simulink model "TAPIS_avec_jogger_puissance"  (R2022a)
settings: Solver=ode23t  StartTime=0.0  StopTime=30  RelTol=1e-3  EnableMultiTasking=on
libraries: fl_lib x15, nesl_utility x8, fl_ps_legacy_lib x1, simulink x1, ee_lib x1

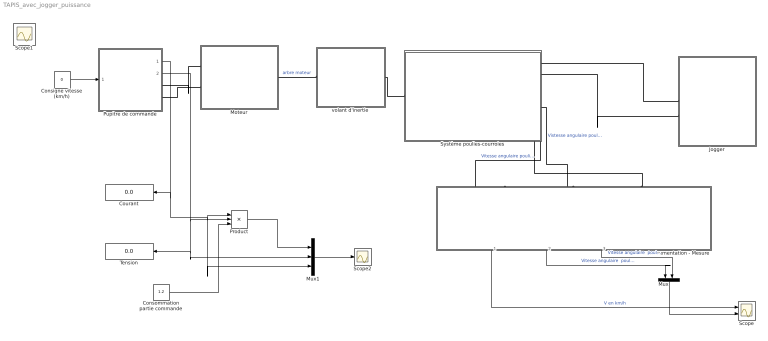
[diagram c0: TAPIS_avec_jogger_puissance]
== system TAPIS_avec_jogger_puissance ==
  Consigne vitesse (km/h) : Constant  Value=0
  Consommation partie commande : Constant  Value=1.2
  Courant : Display
  Instrumentation - Mesure : Subsystem
  Jogger : Subsystem  mask{m=0}
      mask prompts: m "Masse individu"
  Moteur : Subsystem  mask{R=1.7, L=1.2e-1, Kv=0.0152, J=0.000971, Cs=0.076936, Cv=0.000159}
      mask prompts: R "Résistance R en Ohms"; L "Inductance de l'induit L en Henrys"; Kv "Constante de vitesse Kv en V/tr.min-1"; J "Moment d'inertie du Moteur J en Kg.m²"; Cs "Couple de frottements secs Cs en N.m"; Cv "Couple de frottements visqueux Cv en N.m/(rad/s)"
  Mux : Mux  Inputs=2
  Mux1 : Mux  Inputs=3
  Product : Product  Inputs=3
  Pupitre de commande : Subsystem
  Scope : Scope  NumInputPorts=2
  Scope2 : Scope
  Système poulies-courroies : Subsystem  mask{rapportreduction=3.3, rayonrouleau=0.02075}
      mask prompts: rapportreduction "Rapport de réduction du système poulies-courroie"; rayonrouleau "Rayon du rouleau entrainant r en m"
  Tension : Display
  volant d'inertie : Subsystem  mask{inertie=0.007860}
      mask prompts: inertie "Inertie en kg.m²"
  Scope1 : Scope
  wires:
  Consigne vitesse (km/h)/1 -> Pupitre de commande/1(In1)
  Mux/1 -> Scope/2
  Instrumentation - Mesure/2(Vitesse angulaire poulie menante en rad/s) -> Mux/1  "Vitesse angulaire  poulie menée"
  Instrumentation - Mesure/1(Vitesse linéaire en km/h) -> Scope/1  "V en km/h"
  Instrumentation - Mesure/3(Vitesse angulaire poulie menée en rad/s) -> Mux/2  "Vitesse angulaire  poulie menante"
  Pupitre de commande/1(courant) -> Mux1/3, Product/1, Courant/1
  Pupitre de commande/2(tension) -> Mux1/2, Tension/1, Product/2
  Mux1/1 -> Scope2/1
  Product/1 -> Mux1/1
  Consommation partie commande/1 -> Product/3
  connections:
  Moteur/LConn1 -- Pupitre de commande/RConn1
  volant d'inertie/LConn1 -- Moteur/RConn1  "arbre moteur"
  Système poulies-courroies/RConn6 -- Instrumentation - Mesure/LConn1  "Vitesse angulaire poulie menée"
  Système poulies-courroies/RConn5 -- Instrumentation - Mesure/LConn2  "Vistesse angulaire poulie menante"
  Instrumentation - Mesure/LConn3 -- Système poulies-courroies/RConn3
  volant d'inertie/RConn1 -- Système poulies-courroies/LConn1
  Pupitre de commande/RConn2 -- Moteur/LConn2
  Système poulies-courroies/RConn1 -- Jogger/LConn1
  Système poulies-courroies/RConn2 -- Jogger/LConn2

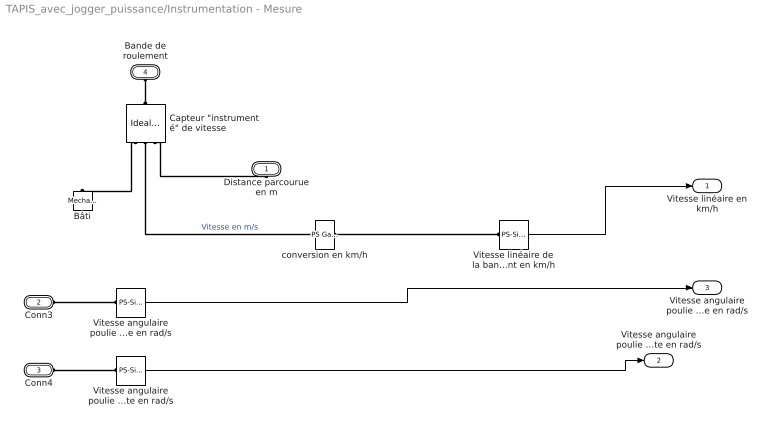
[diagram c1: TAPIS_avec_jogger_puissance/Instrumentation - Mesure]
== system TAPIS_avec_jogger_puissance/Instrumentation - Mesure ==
  Bâti : fl_lib/Mechanical/Translational Elements/Mechanical Translational Reference
  "Capteur \"instrumenté\" de vitesse" : fl_lib/Mechanical/Mechanical Sensors/Ideal Translational Motion Sensor  offset=0 m
  Vitesse angulaire poulie menante en rad/s : nesl_utility/PS-Simulink Converter  PhysicalDomain=network_engine_domain  SubClassName=ps_output  LeftPortType=input  RightPortType=output  PseudoPeriodic=off  Frequencies=[]  VectorFormat=1-D array  Unit=rad/s  AffineConversion=off
  Vitesse angulaire poulie menée en rad/s : nesl_utility/PS-Simulink Converter  PhysicalDomain=network_engine_domain  SubClassName=ps_output  LeftPortType=input  RightPortType=output  PseudoPeriodic=off  Frequencies=[]  VectorFormat=1-D array  Unit=rad/s  AffineConversion=off
  Vitesse linéaire de la bande de roulement en km/h : nesl_utility/PS-Simulink Converter  PhysicalDomain=network_engine_domain  SubClassName=ps_output  LeftPortType=input  RightPortType=output  PseudoPeriodic=off  Frequencies=[]  VectorFormat=1-D array  Unit=1  AffineConversion=off
  conversion en km/h : fl_ps_legacy_lib/Legacy Physical Signals/Functions/PS Gain  gain=3.6
  Distance parcourue en m : PMIOPort  Side=Right
  Conn3 : PMIOPort  Port=2  Side=Left
  Conn4 : PMIOPort  Port=3  Side=Left
  Bande de roulement : PMIOPort  Port=4  Side=Left
  Vitesse linéaire en km/h : Outport
  Vitesse angulaire poulie menante en rad/s : Outport  Port=2
  Vitesse angulaire poulie menée en rad/s : Outport  Port=3
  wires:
  Vitesse linéaire de la bande de roulement en km/h/1 -> Vitesse linéaire en km/h/1
  Vitesse angulaire poulie menée en rad/s/1 -> Vitesse angulaire poulie menée en rad/s/1
  Vitesse angulaire poulie menante en rad/s/1 -> Vitesse angulaire poulie menante en rad/s/1
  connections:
  Bâti/LConn1 -- "Capteur \"instrumenté\" de vitesse"/RConn1
  "Capteur \"instrumenté\" de vitesse"/RConn2 -- conversion en km/h/LConn1  "Vitesse en m/s"
  conversion en km/h/RConn1 -- Vitesse linéaire de la bande de roulement en km/h/LConn1
  Bande de roulement/RConn1 -- "Capteur \"instrumenté\" de vitesse"/LConn1
  Distance parcourue en m/RConn1 -- "Capteur \"instrumenté\" de vitesse"/RConn3
  Conn3/RConn1 -- Vitesse angulaire poulie menée en rad/s/LConn1
  Conn4/RConn1 -- Vitesse angulaire poulie menante en rad/s/LConn1

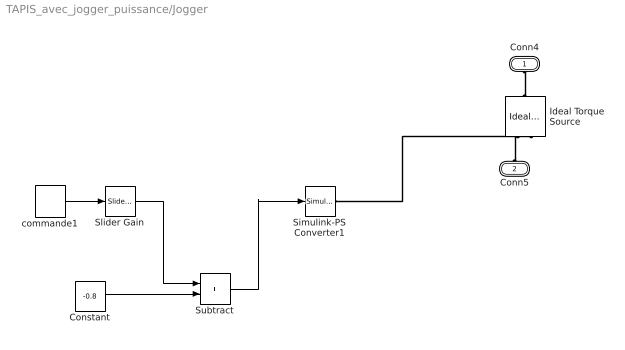
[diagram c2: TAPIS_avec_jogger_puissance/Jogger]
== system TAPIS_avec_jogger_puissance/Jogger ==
  Constant : Constant  Value=-0.8
  Ideal Torque Source : fl_lib/Mechanical/Mechanical Sources/Ideal Torque Source
  Simulink-PS Converter1 : nesl_utility/Simulink-PS Converter  PhysicalDomain=network_engine_domain  SubClassName=ps_input  LeftPortType=input  RightPortType=output  PseudoPeriodic=off  Frequencies=[]  NoiseDistribution=none  NoiseParameters=[]  Unit=N*m  AffineConversion=off  FilteringAndDerivatives=zero  SimscapeFilterOrder=1  InputFilterTimeConstant=.001  UdotUserProvided=0
  Slider Gain : simulink/Math Operations/Slider Gain  gain=17  low=0  high=20
  Subtract : Sum
  commande1 : DiscretePulseGenerator  PulseType=Time based  Amplitude=-m/400  Period=0.4  PulseWidth=50  PhaseDelay=5
  Conn4 : PMIOPort  Side=Left
  Conn5 : PMIOPort  Port=2  Side=Left
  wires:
  Constant/1 -> Subtract/2
  Subtract/1 -> Simulink-PS Converter1/1
  commande1/1 -> Slider Gain/1
  Slider Gain/1 -> Subtract/1
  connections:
  Simulink-PS Converter1/RConn1 -- Ideal Torque Source/RConn1
  Conn4/RConn1 -- Ideal Torque Source/LConn1
  Conn5/RConn1 -- Ideal Torque Source/RConn2

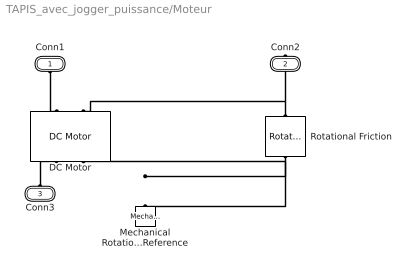
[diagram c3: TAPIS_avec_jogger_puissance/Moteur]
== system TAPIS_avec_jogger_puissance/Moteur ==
  DC Motor : ee_lib/Electromechanical/Brushed Motors/DC Motor  field_option=ee.enum.field_option.pm  Rf=100 Ohm  Lf=1 H  Laf=0.15 H  If0=0 A  parameterization=1  Ra=R Ohm  La=L H  emf_or_torque=1  Kv=Kv V/rpm  Ki=6.876e-4 N*m/A  T_stall=2.4e-4 N*m  w_max=1.91e+4 rpm  w_rated=1.5e+4 rpm  P_rated=0.08 W  V_rated=1.5 V  lam_param=1  i_noload=0 A  V_i_noload=1.5 V  J=0.000971 kg*m^2  lam=0 N*m/(rad/s)  speed0=0 rpm  enable_fault_armature=simscape.enum.onoff.off  rev_faulted=1 / 3  G_faulted_armature=1e-5 S  fault_trigger_armature=ee.enum.faults.faultTrigger.temporal  t_fault_armature=1 s  max_permissible_current_armature=inf A  t_fail_on_current_armature=1 s  enable_fault_field=simscape.enum.onoff.off  G_faulted_field=1e-5 S  fault_trigger_field=ee.enum.faults.faultTrigger.temporal  t_fault_field=1 s  max_permissible_current_field=inf A  t_fail_on_current_field=1 s  fault_action=simscape.enum.assert.action.none  alpha=3.93e-3 1/K  Tmeas=25 degC  thermal_mass=100 J/K  initial_temperature=25 degC
  Mechanical Rotational Reference : fl_lib/Mechanical/Rotational Elements/Mechanical Rotational Reference
  Rotational Friction : fl_lib/Mechanical/Rotational Elements/Rotational Friction  brkwy_trq=Cs*1.25 N*m  brkwy_vel=0.60653 rad/s  Col_trq=Cs N*m  visc_coef=Cv N*m/(rad/s)  w_specify=off  w_priority=None  w=0 rad/s  w_nominal_specify=off  w_nominal_unit=rad/s  w_nominal_value=1  t_specify=off  t_priority=None  t=0 N*m  t_nominal_specify=off  t_nominal_unit=N*m  t_nominal_value=1
  Conn1 : PMIOPort  Side=Left
  Conn2 : PMIOPort  Port=2  Side=Right
  Conn3 : PMIOPort  Port=3  Side=Left
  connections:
  Conn1/RConn1 -- DC Motor/LConn1
  Rotational Friction/LConn1 -- DC Motor/LConn2 -- Conn2/RConn1
  Conn3/RConn1 -- DC Motor/RConn1
  Rotational Friction/RConn1 -- DC Motor/RConn2 -- Mechanical Rotational Reference/LConn1

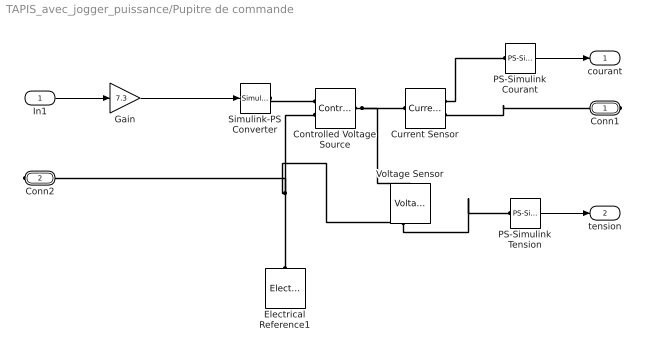
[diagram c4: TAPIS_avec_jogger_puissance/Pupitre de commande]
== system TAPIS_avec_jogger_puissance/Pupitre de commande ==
  In1 : Inport
  Controlled Voltage Source : fl_lib/Electrical/Electrical Sources/Controlled Voltage Source
  Current Sensor : fl_lib/Electrical/Electrical Sensors/Current Sensor
  Electrical Reference1 : fl_lib/Electrical/Electrical Elements/Electrical Reference
  Gain : Gain  Gain=7.3
  PS-Simulink Courant : nesl_utility/PS-Simulink Converter  PhysicalDomain=network_engine_domain  SubClassName=ps_output  LeftPortType=input  RightPortType=output  PseudoPeriodic=off  Frequencies=[]  VectorFormat=1-D array  Unit=1  AffineConversion=off
  PS-Simulink Tension : nesl_utility/PS-Simulink Converter  PhysicalDomain=network_engine_domain  SubClassName=ps_output  LeftPortType=input  RightPortType=output  PseudoPeriodic=off  Frequencies=[]  VectorFormat=1-D array  Unit=1  AffineConversion=off
  Simulink-PS Converter : nesl_utility/Simulink-PS Converter  PhysicalDomain=network_engine_domain  SubClassName=ps_input  LeftPortType=input  RightPortType=output  PseudoPeriodic=off  Frequencies=[]  NoiseDistribution=none  NoiseParameters=[]  Unit=1  AffineConversion=off  FilteringAndDerivatives=zero  SimscapeFilterOrder=1  InputFilterTimeConstant=.001  UdotUserProvided=0
  Voltage Sensor : fl_lib/Electrical/Electrical Sensors/Voltage Sensor
  Conn1 : PMIOPort  Side=Right
  Conn2 : PMIOPort  Port=2  Side=Right
  courant : Outport
  tension : Outport  Port=2
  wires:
  PS-Simulink Courant/1 -> courant/1
  PS-Simulink Tension/1 -> tension/1
  In1/1 -> Gain/1
  Gain/1 -> Simulink-PS Converter/1
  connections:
  Simulink-PS Converter/RConn1 -- Controlled Voltage Source/RConn1
  Electrical Reference1/LConn1 -- Conn2/RConn1 -- Controlled Voltage Source/RConn2 -- Voltage Sensor/RConn2
  Controlled Voltage Source/LConn1 -- Voltage Sensor/LConn1 -- Current Sensor/LConn1
  Current Sensor/RConn2 -- Conn1/RConn1
  Current Sensor/RConn1 -- PS-Simulink Courant/LConn1
  Voltage Sensor/RConn1 -- PS-Simulink Tension/LConn1

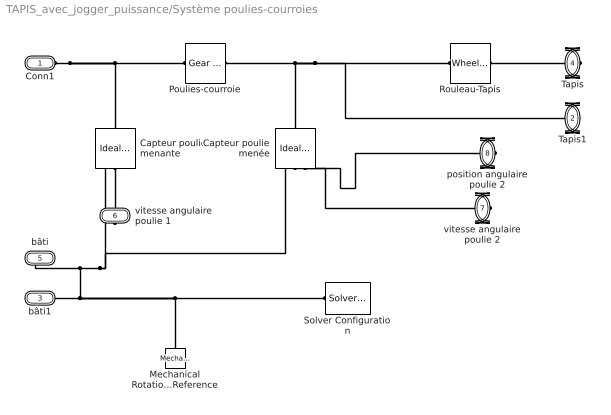
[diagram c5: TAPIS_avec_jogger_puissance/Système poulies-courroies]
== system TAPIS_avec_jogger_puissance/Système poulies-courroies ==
  Capteur poulie menée : fl_lib/Mechanical/Mechanical Sensors/Ideal Rotational Motion Sensor  wrap_angle=simscape.enum.onoff.off  offset=0 rad
  Capteur poulie menante : fl_lib/Mechanical/Mechanical Sensors/Ideal Rotational Motion Sensor  wrap_angle=simscape.enum.onoff.off  offset=0 rad
  Mechanical Rotational Reference : fl_lib/Mechanical/Rotational Elements/Mechanical Rotational Reference
  Poulies-courroie : fl_lib/Mechanical/Mechanisms/Gear Box  ratio=rapportreduction  t_in_specify=off  t_in_priority=None  t_in=0 N*m  t_in_nominal_specify=off  t_in_nominal_unit=N*m  t_in_nominal_value=1  t_out_specify=off  t_out_priority=None  t_out=0 N*m  t_out_nominal_specify=off  t_out_nominal_unit=N*m  t_out_nominal_value=1
  Rouleau-Tapis : fl_lib/Mechanical/Mechanisms/Wheel and Axle  R=rayonrouleau m  or=1  t_specify=off  t_priority=None  t=0 N*m  t_nominal_specify=off  t_nominal_unit=N*m  t_nominal_value=1  f_specify=off  f_priority=None  f=0 N  f_nominal_specify=off  f_nominal_unit=N  f_nominal_value=1
  Solver Configuration : nesl_utility/Solver Configuration  PhysicalDomain=network_engine_domain  SubClassName=solver  LeftPortType=input  RightPortType=generic  Tones=[]  Harmonics=[]  SimulateNoise=off  Profile=off  UseLocalSampling=off  EnableSwitchedLinearOptims=on  FrequencyDomain=off  UseCCode=off  RelTol=0.001  AbsTol=1e-06  MinStep=1e-09  ToWorkspace=off  RevertToSquareIcSolve=off  NumHomotopyIterations=100  PhasorMode=off  PhasorModeNumHarmonics=1  IndexReductionMethod=DerivativeReplacement  DoDC=on  ResidualTolerance=1e-9  UseLocalSolver=off  LocalSolverChoice=NE_BACKWARD_EULER_ADVANCER  LocalSolverSampleTime=.001  DoFixedCost=off  MaxNonlinIter=3  MaxModeIter=2  ComputeImpulses=off  ImpulseIterations=2  LinearAlgebra=Sparse  LinearAlgebraNumThread=0  EquationFormulation=NE_TIME_EF  DelaysMemoryBudget=1024  AutomaticFiltering=on  FilteringTimeConstant=0.001  PartitionStorageMethod=AS_NEEDED  PartitionMemoryBudget=1024  PartitionMethod=FAST
  Conn1 : PMIOPort  Side=Left
  Tapis1 : PMIOPort  Port=2  Side=Right
  bâti1 : PMIOPort  Port=3  Side=Right
  Tapis : PMIOPort  Port=4  Side=Right
  bâti : PMIOPort  Port=5  Side=Right
  vitesse angulaire poulie 1 : PMIOPort  Port=6  Side=Right
  vitesse angulaire poulie 2 : PMIOPort  Port=7  Side=Right
  position angulaire poulie 2 : PMIOPort  Port=8  Side=Right
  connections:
  Conn1/RConn1 -- Capteur poulie menante/LConn1 -- Poulies-courroie/LConn1
  Capteur poulie menée/LConn1 -- Poulies-courroie/RConn1 -- Rouleau-Tapis/LConn1 -- Tapis1/RConn1
  vitesse angulaire poulie 1/RConn1 -- Capteur poulie menante/RConn2
  Mechanical Rotational Reference/LConn1 -- Solver Configuration/RConn1 -- bâti/RConn1 -- Capteur poulie menante/RConn1 -- Capteur poulie menée/RConn1 -- bâti1/RConn1
  Tapis/RConn1 -- Rouleau-Tapis/RConn1
  vitesse angulaire poulie 2/RConn1 -- Capteur poulie menée/RConn2
  position angulaire poulie 2/RConn1 -- Capteur poulie menée/RConn3

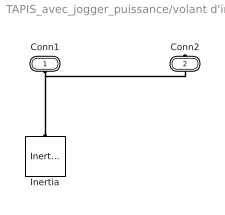
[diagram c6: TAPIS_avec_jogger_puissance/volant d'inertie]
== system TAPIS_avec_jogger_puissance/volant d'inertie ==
  Inertia : fl_lib/Mechanical/Rotational Elements/Inertia  inertia=inertie kg*m^2  num_ports=foundation.enum.numPorts2.one  w_specify=on  w_priority=High  w=0 rad/s  w_nominal_specify=off  w_nominal_unit=rad/s  w_nominal_value=1  t_specify=off  t_priority=None  t=0 N*m  t_nominal_specify=off  t_nominal_unit=N*m  t_nominal_value=1
  Conn1 : PMIOPort  Side=Left
  Conn2 : PMIOPort  Port=2  Side=Right
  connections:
  Conn1/RConn1 -- Conn2/RConn1 -- Inertia/LConn1
